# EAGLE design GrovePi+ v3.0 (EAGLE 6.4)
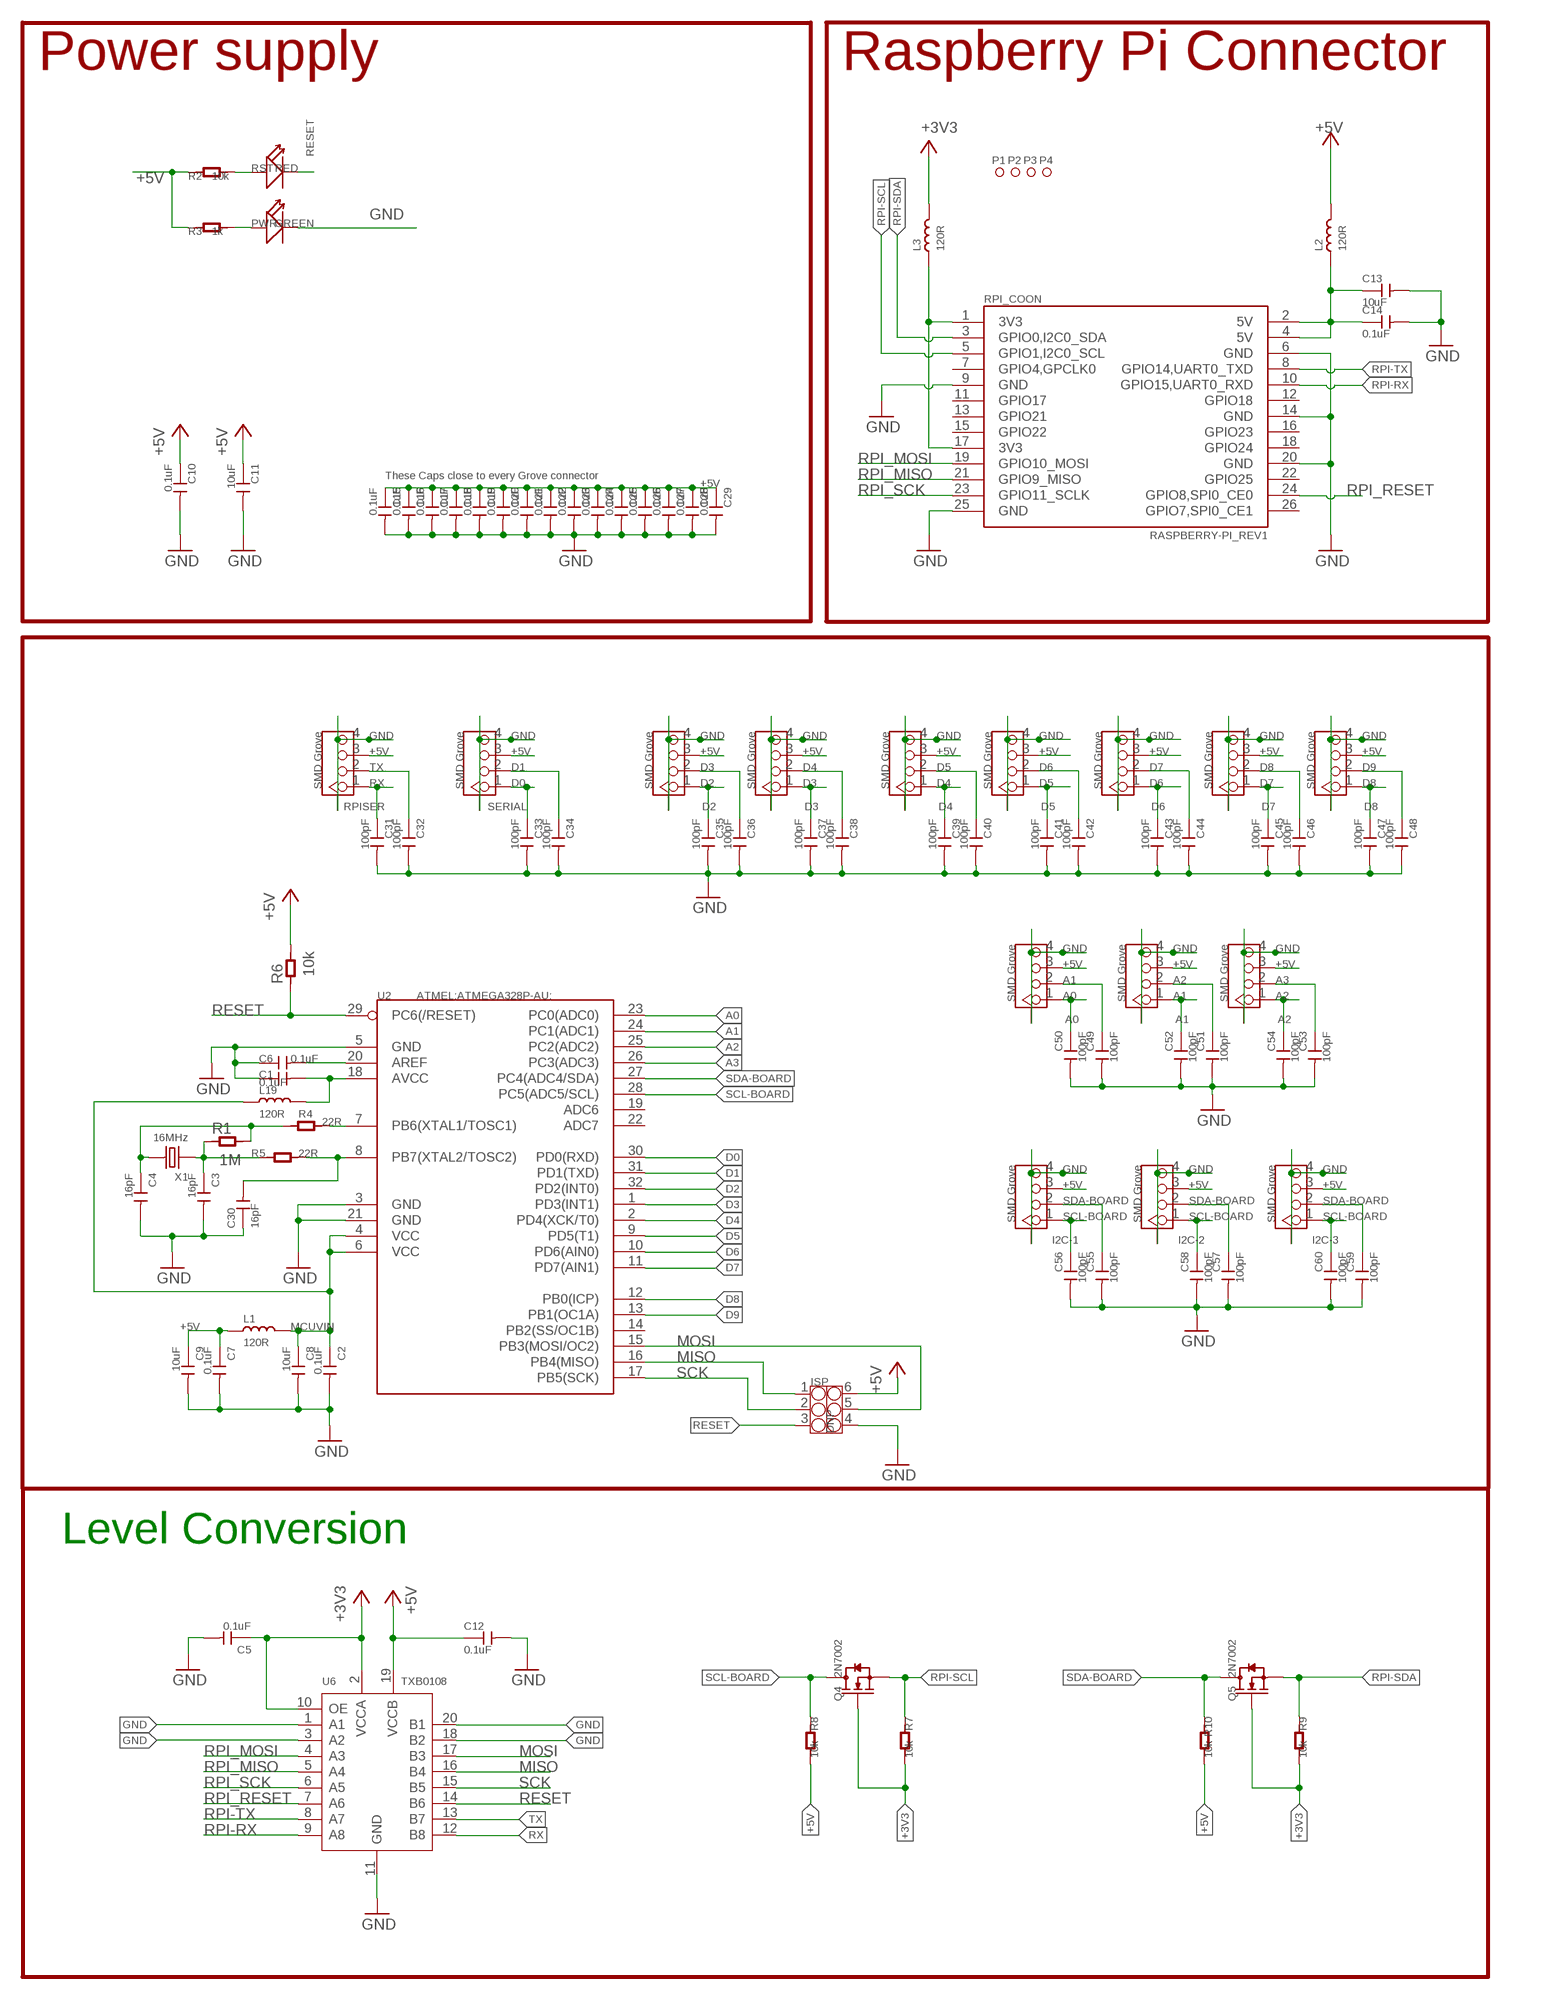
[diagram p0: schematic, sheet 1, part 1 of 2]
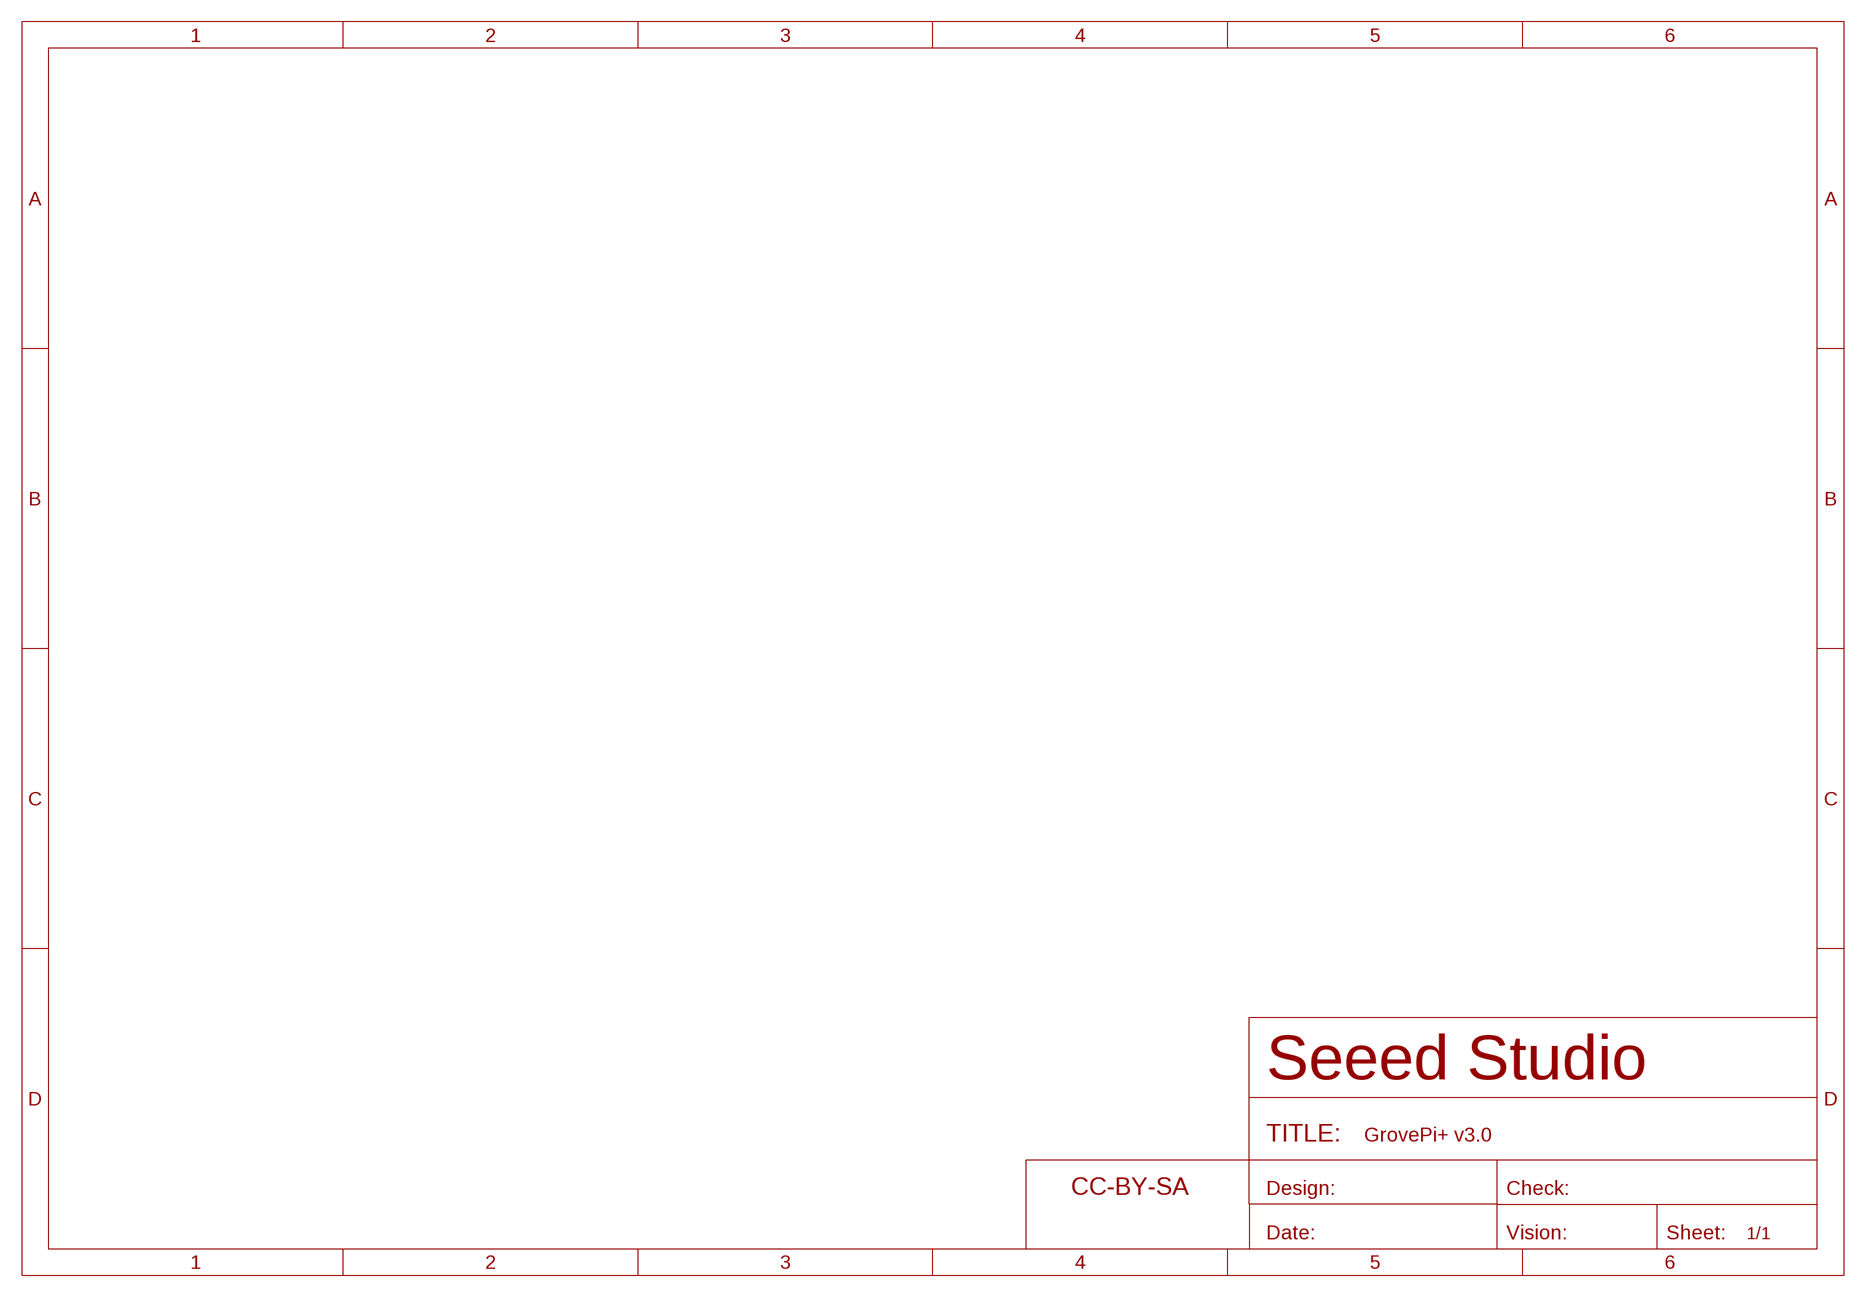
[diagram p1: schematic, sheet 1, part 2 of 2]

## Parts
A0  SMD Grove  GROVE-CONNECTOR-SMD'90D'  [HW4-SMD-2.0-90D]
A1  SMD Grove  GROVE-CONNECTOR-SMD'90D'  [HW4-SMD-2.0-90D]
A2  SMD Grove  GROVE-CONNECTOR-SMD'90D'  [HW4-SMD-2.0-90D]
C1  0.1uF  CAP-0603  [C0603]
C2  0.1uF  CAP-0603  [C0603]
C3  16pF  CAP-0603  [C0603]
C4  16pF  CAP-0603  [C0603]
C5  0.1uF  CAP-0603  [C0603]
C6  0.1uF  CAP-0603  [C0603]
C7  0.1uF  CAP-0603  [C0603]
C8  10uF  CAP-0805  [C0805]
C9  10uF  CAP-0805  [C0805]
C10  0.1uF  CAP-0603  [C0603]
C11  10uF  CAP-0805  [C0805]
C12  0.1uF  CAP-0603  [C0603]
C13  10uF  CAP-0805  [C0805]
C14  0.1uF  CAP-0603  [C0603]
C15  0.1uF  CAP-0603  [C0603]
C16  0.1uF  CAP-0603  [C0603]
C17  0.1uF  CAP-0603  [C0603]
C18  0.1uF  CAP-0603  [C0603]
C19  0.1uF  CAP-0603  [C0603]
C20  0.1uF  CAP-0603  [C0603]
C21  0.1uF  CAP-0603  [C0603]
C22  0.1uF  CAP-0603  [C0603]
C23  0.1uF  CAP-0603  [C0603]
C24  0.1uF  CAP-0603  [C0603]
C25  0.1uF  CAP-0603  [C0603]
C26  0.1uF  CAP-0603  [C0603]
C27  0.1uF  CAP-0603  [C0603]
C28  0.1uF  CAP-0603  [C0603]
C29  0.1uF  CAP-0603  [C0603]
C30  16pF  CAP-0402  [C0402]
C31  100pF  CAP-0603  [C0603]
C32  100pF  CAP-0603  [C0603]
C33  100pF  CAP-0603  [C0603]
C34  100pF  CAP-0603  [C0603]
C35  100pF  CAP-0603  [C0603]
C36  100pF  CAP-0603  [C0603]
C37  100pF  CAP-0603  [C0603]
C38  100pF  CAP-0603  [C0603]
C39  100pF  CAP-0603  [C0603]
C40  100pF  CAP-0603  [C0603]
C41  100pF  CAP-0603  [C0603]
C42  100pF  CAP-0603  [C0603]
C43  100pF  CAP-0603  [C0603]
C44  100pF  CAP-0603  [C0603]
C45  100pF  CAP-0603  [C0603]
C46  100pF  CAP-0603  [C0603]
C47  100pF  CAP-0603  [C0603]
C48  100pF  CAP-0603  [C0603]
C49  100pF  CAP-0603  [C0603]
C50  100pF  CAP-0603  [C0603]
C51  100pF  CAP-0603  [C0603]
C52  100pF  CAP-0603  [C0603]
C53  100pF  CAP-0603  [C0603]
C54  100pF  CAP-0603  [C0603]
C55  100pF  CAP-0603  [C0603]
C56  100pF  CAP-0603  [C0603]
C57  100pF  CAP-0603  [C0603]
C58  100pF  CAP-0603  [C0603]
C59  100pF  CAP-0603  [C0603]
C60  100pF  CAP-0603  [C0603]
D2  SMD Grove  GROVE-CONNECTOR-SMD'90D'  [HW4-SMD-2.0-90D]
D3  SMD Grove  GROVE-CONNECTOR-SMD'90D'  [HW4-SMD-2.0-90D]
D4  SMD Grove  GROVE-CONNECTOR-SMD'90D'  [HW4-SMD-2.0-90D]
D5  SMD Grove  GROVE-CONNECTOR-SMD'DD'  [HW4-SMD-2.0]
D6  SMD Grove  GROVE-CONNECTOR-SMD'DD'  [HW4-SMD-2.0]
D7  SMD Grove  GROVE-CONNECTOR-SMD'90D'  [HW4-SMD-2.0-90D]
D8  SMD Grove  GROVE-CONNECTOR-SMD'90D'  [HW4-SMD-2.0-90D]
I2C-1  SMD Grove  GROVE-CONNECTOR-SMD'90D'  [HW4-SMD-2.0-90D]
I2C-2  SMD Grove  GROVE-CONNECTOR-SMD'90D'  [HW4-SMD-2.0-90D]
I2C-3  SMD Grove  GROVE-CONNECTOR-SMD'90D'  [HW4-SMD-2.0-90D]
ISP  DNP  CONNECTOR-HEADER-2X3P-3460180P1  [2X3P-2.54-2.54-11.6-3.0-BLACK-MALE]
L1  120R  INDUCTOR/FERRITE-BEAD'0603'  [L0603]
L2  120R  INDUCTOR/FERRITE-BEAD'0603'  [L0603]
L3  120R  INDUCTOR/FERRITE-BEAD'0603'  [L0603]
L19  120R  INDUCTOR/FERRITE-BEAD'0603'  [L0603]
P1  PAD-MARK'ANNULAR'  [ROUND-MARK-1.0]
P2  PAD-MARK'ANNULAR'  [ROUND-MARK-1.0]
P3  PAD-MARK'ANNULAR'  [ROUND-MARK-1.0]
P4  PAD-MARK'ANNULAR'  [ROUND-MARK-1.0]
PWR  GREEN  LED  [LED0603]
Q4  2N7002  MOSFET-N-''  [SOT23]
Q5  2N7002  MOSFET-N-''  [SOT23]
R1  1M  R-0402  [R0402]
R2  10k  R-0603  [R0603]
R3  1k  R-0603  [R0603]
R4  22R  R-0402  [R0402]
R5  22R  R-0402  [R0402]
R6  10k  R-0603  [R0603]
R7  10k  R-0603  [R0603]
R8  10k  R-0603  [R0603]
R9  10k  R-0603  [R0603]
R10  10k  R-0603  [R0603]
RPI_COON  RASPBERRY-PI_REV1  [RASPBERRY-PI_REV1]
RPISER  SMD Grove  GROVE-CONNECTOR-SMD'90D'  [HW4-SMD-2.0-90D]
RST  RED  LED  [LED0603]
SERIAL  SMD Grove  GROVE-CONNECTOR-SMD'90D'  [HW4-SMD-2.0-90D]
U2  ATMEL;ATMEGA328P-AU;  ATMEGA328P-AU-1030060P1  [TQFP32]
U6  TXB0108  TXS0108E  [TSSOP20]
U$4  SEEEDSTUDIO-OPEN-SCH-FRAME  [SEEEDSTUDIO-PCB-FRAME]
X1  16MHz  CRYSTAL-2P'5032'  [X2-SMD-5.0X3.2X1.3MM]

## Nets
+3V3: C5.1 L3.2 Q4.1(G) Q5.1(G) R7.2 R9.2 U6.2(VCCA) U6.10(OE)
+5V: A0.3 A1.3 A2.3 C7.1 C9.1 C10.1 C11.1 C12.1 C15.1 C16.1 C17.1 C18.1 C19.1 C20.1 C21.1 C22.1 C23.1 C24.1 C25.1 C26.1 C27.1 C28.1 C29.1 D2.3 D3.3 D4.3 D5.3 D6.3 D7.3 D8.3 I2C-1.3 I2C-2.3 I2C-3.3 ISP.6 L1.1 L2.2 R2.1 R3.1 R6.2 R8.2 R10.2 RPISER.3 SERIAL.3 U6.19(VCCB)
A0: A0.1 C50.1 U2.23(PC0(ADC0))
A1: A0.2 A1.1 C49.1 C52.1 U2.24(PC1(ADC1))
A2: A1.2 A2.1 C51.1 C54.1 U2.25(PC2(ADC2))
A3: A2.2 C53.1 U2.26(PC3(ADC3))
D0: C33.1 SERIAL.1 U2.30(PD0(RXD))
D1: C34.1 SERIAL.2 U2.31(PD1(TXD))
D2: C35.1 D2.1 U2.32(PD2(INT0))
D3: C36.1 C37.1 D2.2 D3.1 U2.1(PD3(INT1))
D4: C38.1 C39.1 D3.2 D4.1 U2.2(PD4(XCK/T0))
D5: C40.1 C41.1 D4.2 D5.1 U2.9(PD5(T1))
D6: C42.1 C43.1 D5.2 D6.1 U2.10(PD6(AIN0))
D7: C44.1 C45.1 D6.2 D7.1 U2.11(PD7(AIN1))
D8: C46.1 C47.1 D7.2 D8.1 U2.12(PB0(ICP))
D9: C48.1 D8.2 U2.13(PB1(OC1A))
GND: A0.4 A0.SS1 A0.SS2 A1.4 A1.SS1 A1.SS2 A2.4 A2.SS1 A2.SS2 C1.1 C2.2 C3.2 C4.2 C5.2 C6.1 C7.2 C8.2 C9.2 C10.2 C11.2 C12.2 C13.2 C14.2 C15.2 C16.2 C17.2 C18.2 C19.2 C20.2 C21.2 C22.2 C23.2 C24.2 C25.2 C26.2 C27.2 C28.2 C29.2 C30.1 C31.2 C32.2 C33.2 C34.2 C35.2 C36.2 C37.2 C38.2 C39.2 C40.2 C41.2 C42.2 C43.2 C44.2 C45.2 C46.2 C47.2 C48.2 C49.2 C50.2 C51.2 C52.2 C53.2 C54.2 C55.2 C56.2 C57.2 C58.2 C59.2 C60.2 D2.4 D2.SS1 D2.SS2 D3.4 D3.SS1 D3.SS2 D4.4 D4.SS1 D4.SS2 D5.4 D5.SS1 D5.SS2 D6.4 D6.SS1 D6.SS2 D7.4 D7.SS1 D7.SS2 D8.4 D8.SS1 D8.SS2 I2C-1.4 I2C-1.SS1 I2C-1.SS2 I2C-2.4 I2C-2.SS1 I2C-2.SS2 I2C-3.4 I2C-3.SS1 I2C-3.SS2 ISP.4 PWR.- RPI_COON.6(GND) RPI_COON.9(GND) RPI_COON.14(GND) RPI_COON.20(GND) RPI_COON.25(GND) RPISER.4 RPISER.SS1 RPISER.SS2 SERIAL.4 SERIAL.SS1 SERIAL.SS2 U2.3(GND) U2.5(GND) U2.21(GND) U6.1(A1) U6.3(A2) U6.11(GND) U6.18(B2) U6.20(B1)
MCUVIN: C2.1 C8.1 L1.2 L19.1 U2.4(VCC) U2.6(VCC)
MISO: ISP.1 U2.16(PB4(MISO)) U6.16(B4)
MOSI: ISP.5 U2.15(PB3(MOSI/OC2)) U6.17(B3)
N$1: C3.1 R1.1 R5.1 X1.1
N$2: PWR.+ R3.2
N$3: C4.1 R1.2 R4.1 X1.2
N$4: C1.2 L19.2 U2.18(AVCC)
N$17: R2.2 RST.+
N$19: L3.1 RPI_COON.1(3V3) RPI_COON.17(3V3)
N$20: C6.2 U2.20(AREF)
N$21: C13.1 C14.1 L2.1 RPI_COON.2(5V) RPI_COON.4(5V)
N$22: C30.2 R5.2 U2.8(PB7(XTAL2/TOSC2))
N$23: R4.2 U2.7(PB6(XTAL1/TOSC1))
RESET: ISP.3 R6.1 RST.- U2.29(PC6(/RESET)) U6.14(B6)
RPI-RX: RPI_COON.10(GPIO15,UART0_RXD) U6.9(A8)
RPI-SCL: Q4.2(S) R7.1 RPI_COON.5(GPIO1,I2C0_SCL)
RPI-SDA: Q5.2(S) R9.1 RPI_COON.3(GPIO0,I2C0_SDA)
RPI-TX: RPI_COON.8(GPIO14,UART0_TXD) U6.8(A7)
RPI_MISO: RPI_COON.21(GPIO9_MISO) U6.5(A4)
RPI_MOSI: RPI_COON.19(GPIO10_MOSI) U6.4(A3)
RPI_RESET: RPI_COON.24(GPIO8,SPI0_CE0) U6.7(A6)
RPI_SCK: RPI_COON.23(GPIO11_SCLK) U6.6(A5)
RX: C31.1 RPISER.1 U6.12(B8)
SCK: ISP.2 U2.17(PB5(SCK)) U6.15(B5)
SCL-BOARD: C56.1 C58.1 C60.1 I2C-1.1 I2C-2.1 I2C-3.1 Q4.3(D) R8.1 U2.28(PC5(ADC5/SCL))
SDA-BOARD: C55.1 C57.1 C59.1 I2C-1.2 I2C-2.2 I2C-3.2 Q5.3(D) R10.1 U2.27(PC4(ADC4/SDA))
TX: C32.1 RPISER.2 U6.13(B7)
Unconnected: RPI_COON.7(GPIO4,GPCLK0) RPI_COON.11(GPIO17) RPI_COON.12(GPIO18) RPI_COON.13(GPIO21) RPI_COON.15(GPIO22) RPI_COON.16(GPIO23) RPI_COON.18(GPIO24) RPI_COON.22(GPIO25) RPI_COON.26(GPIO7,SPI0_CE1) U2.14(PB2(SS/OC1B)) U2.19(ADC6) U2.22(ADC7)

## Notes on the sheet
- Power supply | Raspberry Pi Connector
- These Caps close to every Grove connector
- Level Conversion

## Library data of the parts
A0 A1 A2 D2-D8 I2C-1-I2C-3 RPISER SERIAL = Connector-new:GROVE-CONNECTOR-SMD: 4P-SMD-2.0:320110030;4P-SMD-2.0-90D:320110032
C1-C60 = OPL:CAP: Ceramic Capacitors
ISP = OPL:CONNECTOR-HEADER-2X3P
L1-L3 L19 = Discrete-new:INDUCTOR/FERRITE-BEAD
P1-P4 = Discrete-new:PAD-MARK; PARTNO: DNP
PWR RST = OPL:LED*: LED
Q4 Q5 = OPL:MOSFET-N: CJ2302：SMD MOSFET N-CH 20V-2.1A
R1-R10 = OPL:R*
RPI_COON = RaspberryPi:RASPBERRY-PI_REV1: Raspberry Pi Board Jacques Lagnel V1.0 (beta) 2012 Mateusz Bawaj V1.1 (beta) 2012 Board dimension: Forum 3D model The GPIO Connector (P1): http://elinux.org/RPi_Low-level_peripherals
U2 = OPL:ATMEGA328P-AU: 8-bit AVR Microcontroller with 32K Bytes In-System Programmable Flash
U6 = template:TXS0108E: 8-BIT BIDIRECTIONAL VOLTAGE-LEVEL TRANSLATOR FOR OPEN-DRAIN AND PUSH-PULL APPLICATIONS
U$4 = moudle-new:SEEEDSTUDIO-OPEN-SCH-FRAME
X1 = Discrete-new:CRYSTAL-2P

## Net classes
0 default: width 0.203 mm
2 POWER: width 0.152 mm, drill 0.356 mm, clearance 0.051 mm

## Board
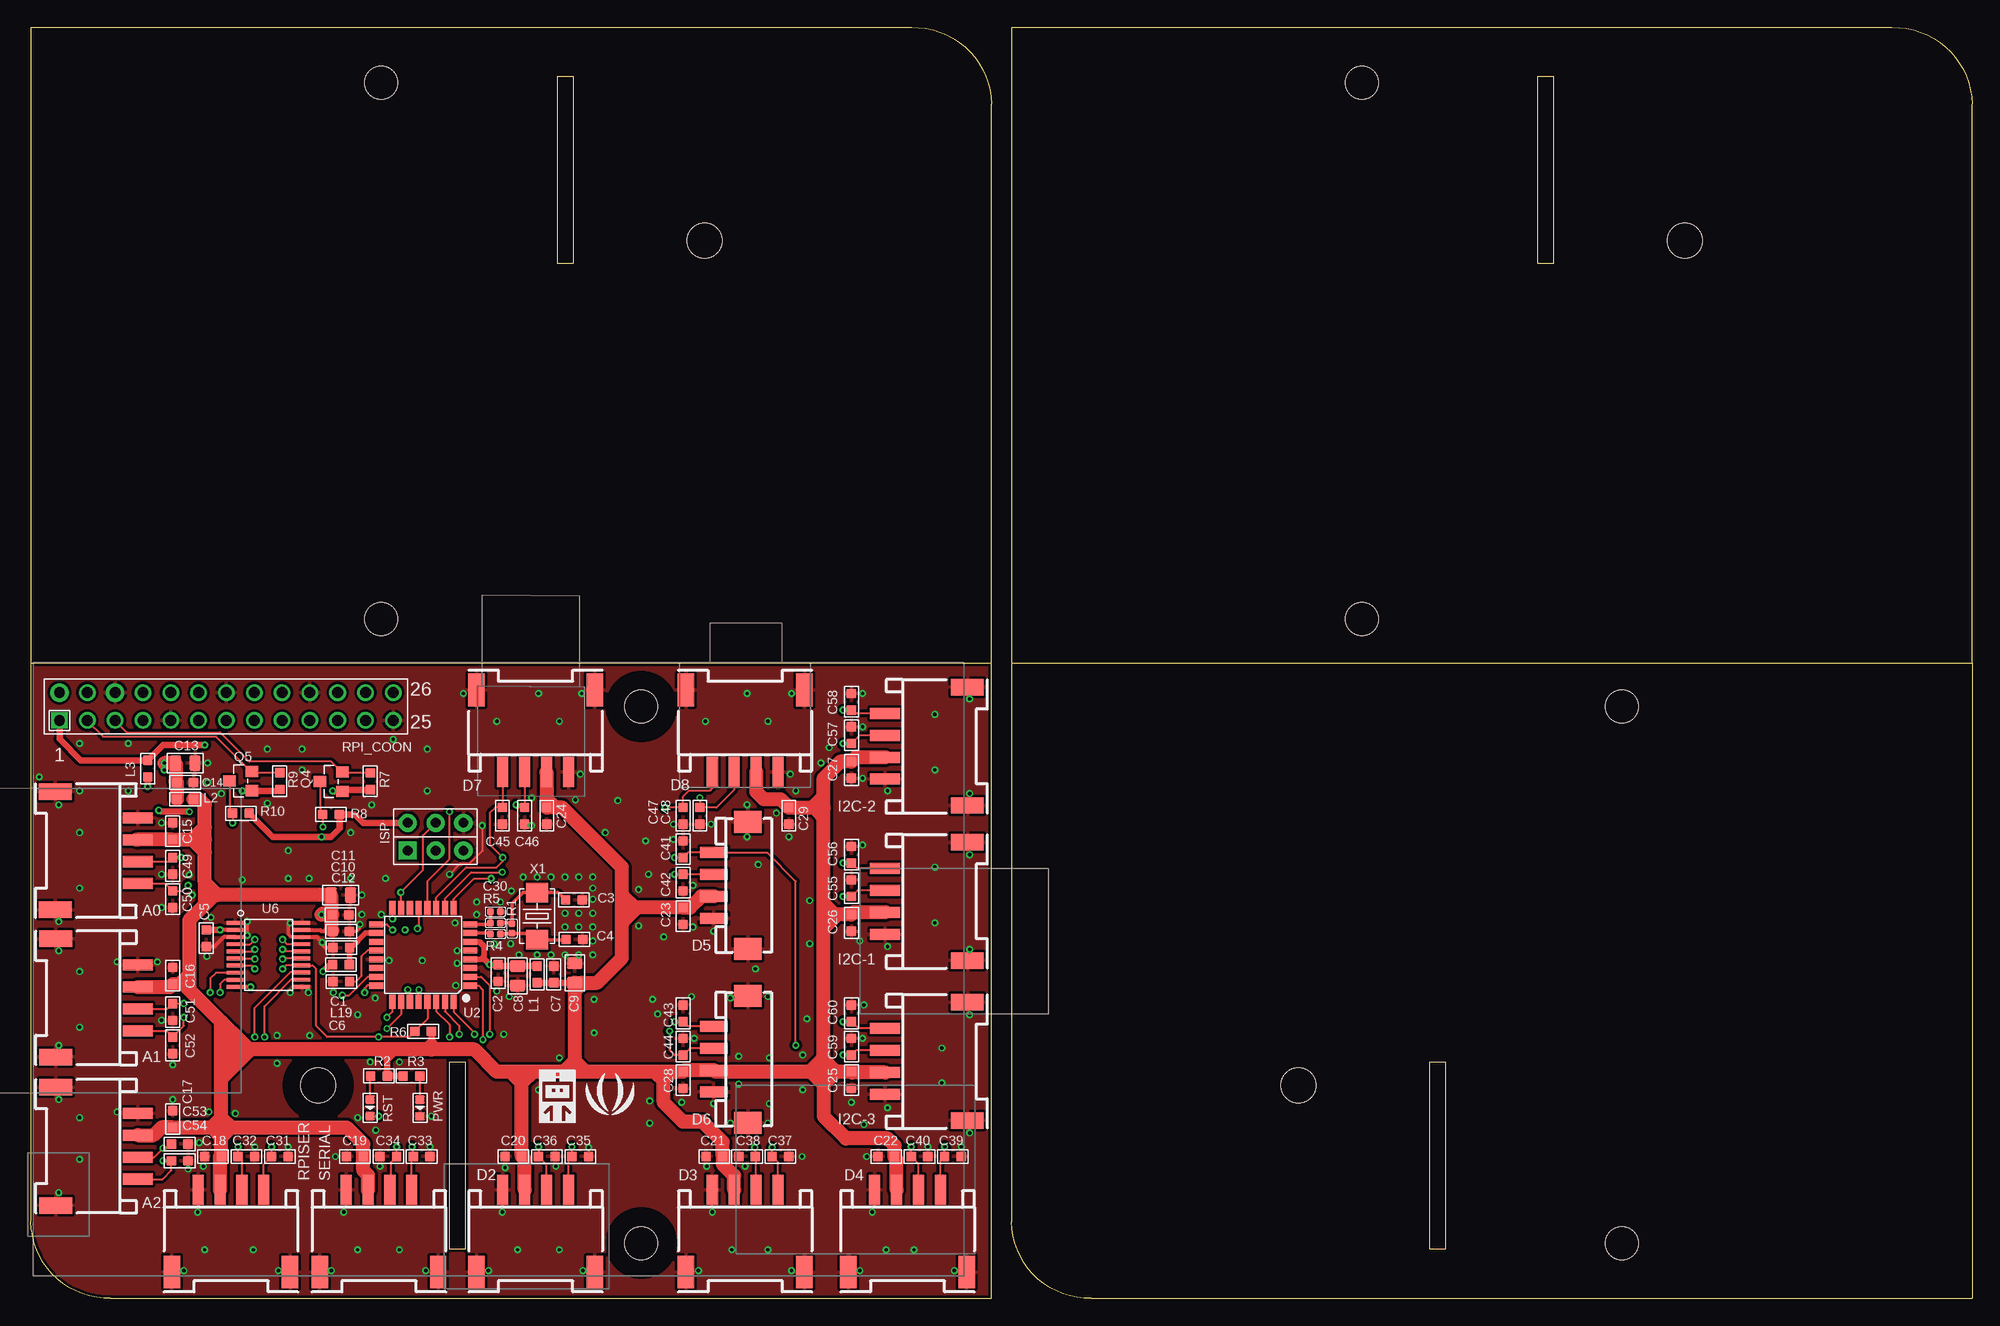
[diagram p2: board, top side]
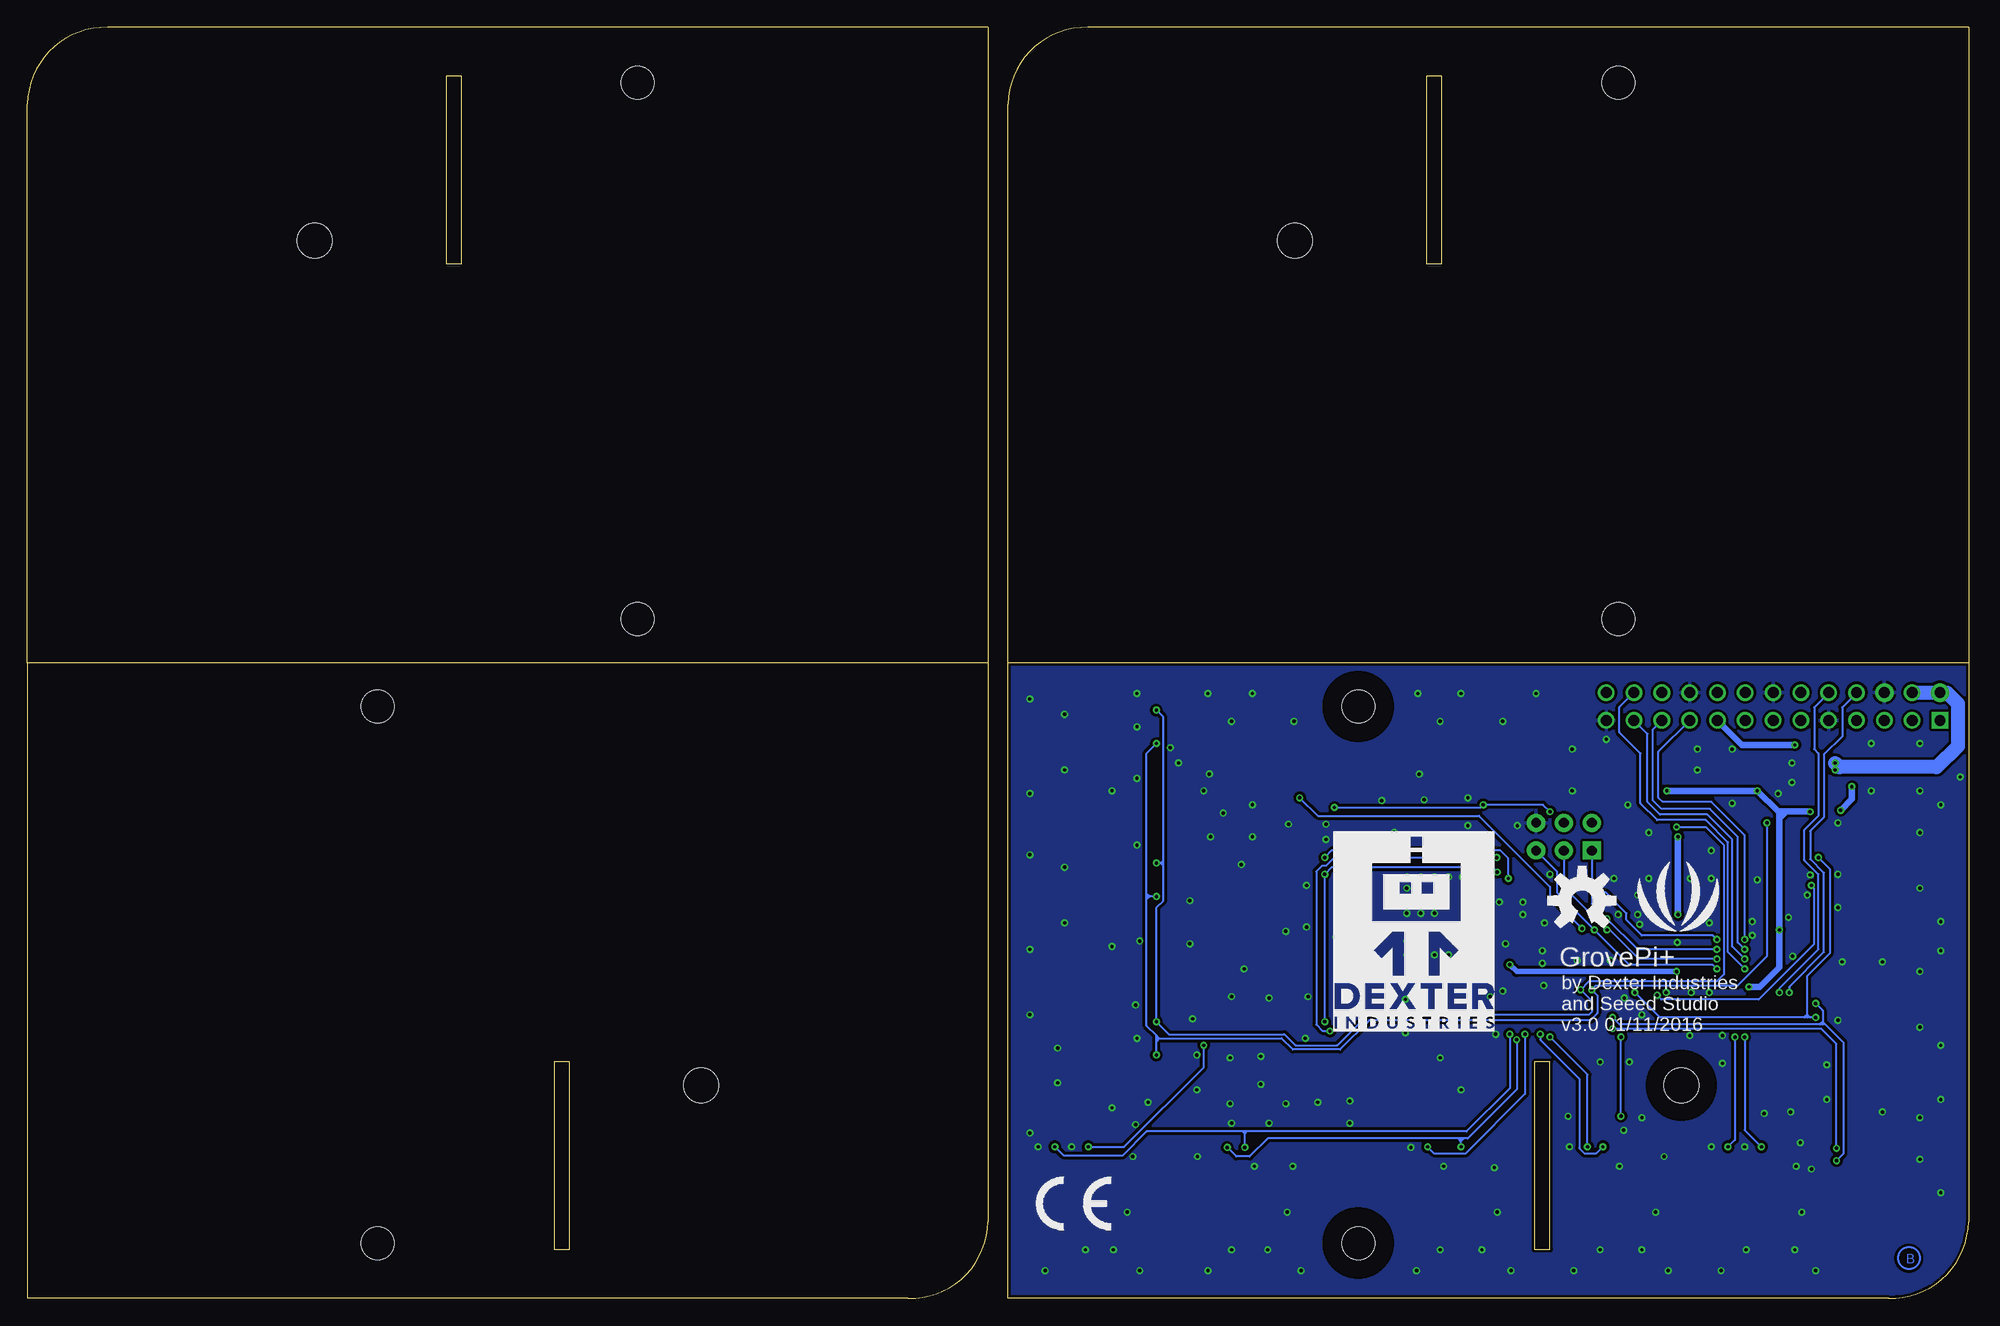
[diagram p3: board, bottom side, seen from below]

Size 177.27 x 116.08 mm. Coordinates in mm from the lower left corner, seen from the top.
Outline: 87.73,58.04 87.73,0 7.32,0 arc-90 0,7.01 0,58.04
Outline: 89.53,58.04 177.27,58.04
Outline: 177.27,58.04 177.27,109.07 arc90 169.95,116.08 89.53,116.08 89.53,58.04
Outline: 0,58.04 0,116.08 80.42,116.08 arc-90 87.73,109.07 87.73,58.04
Outline: 0,58.04 87.73,58.04
Outline: 89.53,58.04 89.53,7.01 arc90 96.85,0 177.27,0 177.27,58.04
Outline: 38.23,21.59 39.65,21.59 39.65,4.47 38.23,4.47 38.23,21.59
Outline: 139.04,94.49 137.62,94.49 137.62,111.61 139.04,111.61 139.04,94.49
Outline: 49.51,94.49 48.08,94.49 48.08,111.61 49.51,111.61 49.51,94.49
Outline: 127.76,21.59 129.18,21.59 129.18,4.47 127.76,4.47 127.76,21.59
Copper layers (1*16): Top 0.035mm / dielectric 1.5mm / Bottom 0.035mm
Design rules "SeeedStudio_2layer_DRU_no_angle_20140221 *": minimum track width 6mil, minimum drill 12mil, track to track 6mil, track to pad 6mil, pad to pad 6mil, via to via 6mil, smd to smd 0mil, copper to edge 10mil, drill to drill 10mil, minimum pad ring 10mil, minimum via ring 6mil, stop-mask expansion 2mil, vias tented up to drill 25mil, thermal gap 10mil
Holes 3.2 mm at 26.23,19.46 151.04,96.62 61.51,96.62 115.76,19.46
Holes 3 mm at 55.73,54.05 55.73,5.05 121.53,62.03 121.53,111.03 32,62.03 32,111.03 145.27,54.05 145.27,5.05
Holes 2.03 mm at 2.54,-4.45 2.54,120.65 174.62,120.65 174.65,-4.45
tRestrict: area 23.2,16.5 to 29.2,22.5; area 52.7,2 to 58.7,8; area 52.7,51.1 to 58.7,57.1
bRestrict: area 52.7,2 to 58.7,8; area 23.2,16.5 to 29.2,22.5; area 52.7,51.1 to 58.7,57.1

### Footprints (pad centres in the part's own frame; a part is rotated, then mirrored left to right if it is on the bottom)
HW4-SMD-2.0-90D = smd 1.01 x 2.74: 1 -3,-0.1; 2 -1,-0.1; 3 1,-0.1; 4 3,-0.1 | smd 1.5 x 3: SS1 -5.4,7.4; SS2 5.4,7.4
C0603 = smd 0.889 x 0.889: 1 -0.762,0; 2 0.762,0
C0805 = smd 1.016 x 1.397: 1 -0.889,0; 2 0.889,0
C0402 = smd 0.635 x 0.635: 1 -0.445,0; 2 0.445,0
HW4-SMD-2.0 = smd 1 x 2.5: 1 -3,0; 2 -1,0; 3 1,0; 4 3,0 | smd 2 x 2.5: SS1 -5.8,3.123; SS2 5.8,3.123
2X3P-2.54-2.54-11.6-3.0-BLACK-MALE = drill 0.889 pad 1.651 square: 1 -1.27,2.54 | drill 0.889 pad 1.651: 2 -1.27,0; 3 -1.27,-2.54; 4 1.27,-2.54; 5 1.27,0; 6 1.27,2.54
L0603 = smd 0.889 x 0.889: 1 -0.762,0; 2 0.762,0
ROUND-MARK-1.0 = smd 1.016 x 1.016: P$1 0,0
LED0603 = smd 0.762 x 0.889: + -0.762,0; - 0.762,0
SOT23 = smd 1.016 x 1.143: 1 -0.889,-1.016; 2 0.889,-1.016; 3 0,1.016
R0402 = smd 0.635 x 0.635: 1 -0.445,0; 2 0.445,0
R0603 = smd 0.889 x 0.889: 1 -0.762,0; 2 0.762,0
RASPBERRY-PI_REV1 = drill 1 square: 1 -41.91,21.59 | drill 1 pad 1.676: 2 -41.91,24.13; 6 -36.83,24.13 | drill 1: 3 -39.37,21.59; 4 -39.37,24.13; 5 -36.83,21.59; 7 -34.29,21.59; 8 -34.29,24.13; 9 -31.75,21.59; 10 -31.75,24.13; 11 -29.21,21.59; 12 -29.21,24.13; 13 -26.67,21.59; 14 -26.67,24.13; 15 -24.13,21.59; 16 -24.13,24.13; 17 -21.59,21.59; 18 -21.59,24.13; 19 -19.05,21.59; 20 -19.05,24.13; 21 -16.51,21.59; 22 -16.51,24.13; 23 -13.97,21.59; 24 -13.97,24.13; 25 -11.43,21.59; 26 -11.43,24.13
TQFP32 = smd 1.27 x 0.559: 1 -4.293,2.8; 2 -4.293,2; 3 -4.293,1.2; 4 -4.293,0.4; 5 -4.293,-0.4; 6 -4.293,-1.2; 7 -4.293,-2; 8 -4.293,-2.8; 17 4.293,-2.8; 18 4.293,-2; 19 4.293,-1.2; 20 4.293,-0.4; 21 4.293,0.4; 22 4.293,1.2; 23 4.293,2; 24 4.293,2.8 | smd 0.559 x 1.27: 9 -2.8,-4.293; 10 -2,-4.293; 11 -1.2,-4.293; 12 -0.4,-4.293; 13 0.4,-4.293; 14 1.2,-4.293; 15 2,-4.293; 16 2.8,-4.293; 25 2.8,4.293; 26 2,4.293; 27 1.2,4.293; 28 0.4,4.293; 29 -0.4,4.293; 30 -1.2,4.293; 31 -2,4.293; 32 -2.8,4.293
TSSOP20 = smd 0.35 x 1.5: 1 -2.925,-3.065; 2 -2.275,-3.065; 3 -1.625,-3.065; 4 -0.975,-3.065; 5 -0.325,-3.065; 6 0.325,-3.065; 7 0.975,-3.065; 8 1.625,-3.065; 9 2.275,-3.065; 10 2.925,-3.065; 11 2.91,3.065; 12 2.26,3.065; 13 1.61,3.065; 14 0.96,3.065; 15 0.325,3.065; 16 -0.325,3.065; 17 -0.975,3.065; 18 -1.625,3.065; 19 -2.275,3.065; 20 -2.925,3.065
X2-SMD-5.0X3.2X1.3MM = smd 1.778 x 2.032: 1 -2.159,0; 2 2.159,0

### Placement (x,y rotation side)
A0  9.64,40.88 90 top
A1  9.67,27.44 90 top
A2  9.66,13.9 90 top
C1  28.35,32.03 0 top
C2  42.67,29.72 270 top
C3  49.59,36.39 0 top
C4  49.63,32.79 0 top
C5  16.03,32.89 270 top
C6  28.35,28.93 0 top
C7  47.75,29.59 90 top
C8  44.45,29.46 270 top
C9  49.66,29.72 90 top
C10  28.29,35.03 0 top
C11  28.3,36.83 0 top
C12  28.33,33.52 0 top
C13  14.1,48.9 0 top
C14  14.1,47.12 0 top
C15  12.95,42.67 90 top
C16  12.95,29.46 90 top
C17  12.95,16.38 90 top
C18  16.64,12.95 180 top
C19  29.59,12.95 180 top
C20  44.07,12.95 180 top
C21  62.42,12.95 180 top
C22  78.11,12.95 180 top
C23  59.56,34.92 270 top
C24  47.12,44.07 270 top
C25  74.93,19.94 270 top
C26  74.93,34.29 270 top
C27  74.93,48.26 270 top
C28  59.56,19.94 270 top
C29  69.22,44.07 270 top
C30  42.42,35.31 180 top
C31  22.73,12.95 0 top
C32  19.68,12.95 0 top
C33  35.69,12.95 0 top
C34  32.64,12.95 180 top
C35  50.16,12.95 0 top
C36  47.12,12.95 0 top
C37  68.45,12.95 0 top
C38  65.41,12.95 180 top
C39  84.2,12.95 0 top
C40  81.15,12.95 0 top
C41  59.56,41.02 90 top
C42  59.56,37.97 270 top
C43  59.56,26.04 90 top
C44  59.56,22.99 90 top
C45  43.05,44.07 270 top
C46  45.09,44.07 270 top
C47  59.56,44.07 270 top
C48  61.09,44.07 270 top
C49  12.95,39.5 270 top
C50  12.95,36.45 270 top
C51  12.95,26.16 270 top
C52  12.95,23.11 270 top
C53  13.59,14.1 0 top
C54  13.59,12.57 0 top
C55  74.93,37.47 90 top
C56  74.93,40.51 90 top
C57  74.93,51.44 90 top
C58  74.93,54.48 90 top
C59  74.93,22.99 90 top
C60  74.93,26.04 90 top
D2  46.09,9.8 180 top
D3  65.23,9.8 180 top
D4  80.05,9.8 180 top
D5  62.36,37.72 270 top
D6  62.36,21.84 270 top
D7  46.09,48.18 0 top
D8  65.23,48.18 0 top
I2C-1  78.11,36.26 270 top
I2C-2  78.11,50.42 270 top
I2C-3  78.11,21.64 270 top
ISP  36.96,42.16 90 top
L1  46.23,29.59 90 top
L2  14.1,45.59 0 top
L3  10.67,48.39 270 top
L19  28.32,30.48 0 top
P1  not placed on the board
P2  not placed on the board
P3  not placed on the board
P4  not placed on the board
PWR  35.53,17.4 270 top
Q4  27.42,47.2 90 top
Q5  19.17,47.25 90 top
R1  43.94,33.78 270 top
R2  31.8,20.31 180 top
R3  34.76,20.31 0 top
R4  42.42,33.27 180 top
R5  42.42,34.29 180 top
R6  35.82,24.39 0 top
R7  31,47.22 270 top
R8  27.42,44.2 0 top
R9  22.73,47.24 270 top
R10  19.17,44.3 0 top
RPI_COON  44.53,31.19 0 top
RPISER  18.28,9.8 180 top
RST  30.97,17.41 270 top
SERIAL  31.79,9.8 180 top
U2  35.81,31.37 180 top
U6  21.7,31.37 270 top
U$1  [OSHW_FILLX250_NOTEXT]  35.31,36.32 0 bottom
U$2  [SEEED_LOGO250]  30.23,33.53 0 bottom
U$3  [SEEED-LOGO-150]  50.67,16.76 0 top
U$4  not placed on the board
X1  46.23,34.91 270 top

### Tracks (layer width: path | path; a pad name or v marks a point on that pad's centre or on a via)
+3V3  (via drill 0.3 pad 0.64)
  Top 0.356: C5.1 | U6.2 17.28,33.65 v17.27,33.66
  Top 0.406: U6.10 v20.07,28.45 | v20.07,28.45
  Top 0.61: R9.2 22.62,46.36 Q5.1 19.31,46.36 v19.3,46.35 | R7.2 28.58,46.46 Q4.1 27.61,46.31 v27.56,46.35 | C5.1 v17.27,33.65 v17.27,33.66 | v11.68,44.58 11.81,44.45 v14.48,44.45 | L3.2 v10.67,46.74
  Bottom 0.61: v27.56,46.35 v19.3,46.35 17.4,44.45 | 17.4,44.45 17.27,44.32 17.27,43.81 | 17.27,43.81 v17.27,33.66 17.27,30.23 19.05,28.45 v20.07,28.45 | v20.07,28.45 | v11.68,44.58 10.67,45.59 v10.67,46.74 | v14.48,44.45 16.64,44.45 | 16.64,44.45 17.4,44.45 | 16.64,44.45 17.27,43.81
+5V  (via drill 0.3 pad 0.64)
  Top 0.356: U6.19 26.42,33.65 26.55,33.52 C12.1
  Top 0.61: 27.52,33.57 C12.1 | ISP.6 30.35,43.43 29.59,44.2 R8.2 28.18,42.91 27.43,42.16 v26.54,42.16 22.07,42.16 R10.2 | R2.1 R3.1 | 32.64,20.23 R2.1 | 62.56,20.64 D6.3 | R2.1 32.56,21.76 | 32.56,21.8 32.56,22.65 32.64,22.73 | 35.05,22.74 35.05,22.73 | 32.56,21.8 32,22.35 | 32.56,21.76 33.15,22.35 | 32.56,21.76 32.56,21.8 | C9.1 C7.1 L1.1 46.1,28.83 | R6.2 36.58,23.63 | 36.58,23.62 36.58,22.74 36.58,22.73 | 36.58,23.63 35.94,22.99 | 36.58,23.63 36.58,23.62 | 36.58,23.62 37.21,22.99
  Top 1.27: 27.41,35.14 C11.1 17.02,36.83 | 27.41,35.14 C10.1 | 27.41,35.14 27.41,33.68 27.52,33.57 | 27.41,35.14 26.63,35.14 v26.54,35.05 | 16.77,36.83 16,36.83 15.88,36.96 | 15.88,37.97 15.88,36.96 | 15.88,36.96 15.88,35.94 14.48,34.54 14.48,28.7 | 17.02,36.83 16.77,36.83 | 16.77,36.83 16,36.07 | 17.02,36.83 15.88,37.97 | A1.3 12.69,28.44 C16.1 13.59,28.7 | 20.07,22.73 32.64,22.73 35.05,22.73 36.58,22.73 40.51,22.73 42.55,20.7 44.83,20.7 | 20.07,22.73 19.94,22.73 | D2.3 45.09,12.7 C20.1 44.83,19.68 | I2C-2.3 75.33,49.42 C27.1 73.91,49.02 72.39,47.5 72.39,44.83 | D8.3 66.23,46.3 66.93,45.59 68.45,45.59 C29.1 71.37,44.83 | I2C-1.3 75.14,35.26 C26.1 73.66,35.05 | D4.3 79.05,12.64 78.87,12.83 C22.1 78.87,13.97 78.23,14.61 74.42,14.61 72.39,16.64 72.39,19.56 | 15.88,37.97 15.88,40.77 | 15.88,40.77 15.88,41.91 | 15.88,41.91 15.88,43.05 | 15.88,43.05 15.88,45.09 15.37,45.59 L2.2 | 14.73,41.91 C15.1 9.71,41.91 | 14.73,41.91 15.88,41.91 | 9.65,41.91 9.71,41.91 | 9.71,41.91 A0.3 | 14.73,41.91 15.88,43.05 | 14.73,41.91 15.88,40.77 | 14.48,28.7 14.48,28.19 | 14.48,28.19 17.4,25.27 | 17.4,25.27 19.05,23.62 | 19.05,23.62 19.94,22.73 | 13.59,28.7 13.97,28.7 | 13.97,28.7 14.48,28.7 | 14.48,28.19 13.97,28.7 | 13.59,28.7 14.35,29.46 | A2.3 11.21,14.9 11.94,15.62 C17.1 16.51,15.62 | C18.1 17.4,13.08 | 17.4,13.08 17.4,14.73 | 17.4,14.73 17.4,15.62 | 17.4,15.62 17.4,16.51 | 17.4,16.51 17.4,20.07 | 17.4,20.07 17.4,22.73 | 17.4,22.73 17.4,25.27 | 19.94,22.73 17.4,22.73 | 19.05,23.62 18.29,23.62 18.03,23.37 18.03,21.72 18.16,21.59 | 20.07,22.73 17.4,20.07 | 16.51,15.62 17.4,15.62 | 16.51,15.62 17.27,16.38 | 16.51,15.62 17.4,14.73 | RPISER.3 17.27,12.96 17.4,13.08
  Top 1.27: 17.4,15.62 18.29,15.62 | 18.29,15.62 28.83,15.62 30.35,14.1 C19.1 30.35,11.68 30.79,11.25 SERIAL.3 | 58.55,20.7 C28.1 59.71,20.84 D6.3 62.5,20.7 72.39,20.7 | 58.55,20.7 57.78,20.7 | 57.78,20.7 50.67,20.7 | 50.67,20.7 49.66,20.7 | 49.66,20.7 45.85,20.7 | 45.85,20.7 44.83,20.7 | 49.66,28.07 C9.1 50.42,28.83 | 49.66,28.07 49.66,21.72 | 49.66,21.72 49.66,20.7 | 44.83,19.68 44.83,20.7 | 44.83,19.68 43.94,20.57 | 44.83,19.68 45.85,20.7 | 49.66,21.72 48.77,20.83 | 49.66,21.72 50.67,20.7 | D3.3 64.23,11.21 63.18,12.26 C21.1 63.18,14.28 61.34,16.13 59.55,16.13 57.78,17.89 57.78,19.94 | 57.78,19.94 57.78,20.7 | 57.78,19.94 57.15,20.57 | 57.78,19.94 58.55,20.7 | D5.3 61.23,36.72 60.2,35.69 C23.1 55.37,35.69 | 50.42,28.83 51.69,28.83 53.98,31.11 53.98,35.69 | I2C-3.3 74.99,20.64 C25.1 72.39,20.7 | 72.39,21.84 72.39,20.7 | 72.39,21.97 71.25,20.83 | 72.39,21.97 72.39,21.84 | 72.39,21.84 73.41,20.83 | 72.39,21.97 72.39,35.05 | 72.39,35.05 72.39,36.07 | 72.39,36.07 72.39,44.83 | 73.66,35.05 73.41,35.05 | 73.41,35.05 72.39,35.05 | 73.41,35.05 72.39,36.07 | 73.66,35.05 72.52,33.91 | 71.5,44.83 72.39,44.83 | 71.37,44.83 72.14,45.59 | 71.37,44.83 71.5,44.83 | 71.5,44.83 72.14,44.2 | D7.3 47.09,45.62 | 47.09,45.62 47.09,44.86 C24.1 47.88,44.83 | 72.39,20.7 72.39,19.56 | 72.39,19.56 71.37,20.57 | 72.39,19.56 73.28,20.45 | 47.88,44.83 48.51,44.83 53.98,39.37 53.98,35.69 | 47.09,45.62 47.88,44.83 | 50.42,28.83 49.66,28.07 | 17.4,16.51 18.16,15.75 | 18.29,15.62 17.4,14.73 | 55.12,35.69 53.98,35.69 | 55.37,35.69 55.12,35.69 | 55.12,35.69 54.1,36.7 | 55.37,35.69 54.1,34.42
  Bottom 0.61: v26.54,35.05 v26.54,42.16
A0  (via drill 0.3 pad 0.64)
  Top 0.203: U2.23 30.77,29.37 29.08,27.69 v28.45,27.69 | A0.1 12.28,37.88 C50.1 13.84,37.21 v14.35,37.72
  Bottom 0.203: v28.45,27.69 28.07,27.3 19.18,27.3 14.1,32.38 14.1,37.47 v14.35,37.72
A1  (via drill 0.3 pad 0.64)
  Top 0.203: U2.24 30.73,28.57 30.48,28.32 v30.48,27.94 | C49.1 13.08,40.26 | 13.08,40.26 v13.72,40.26 | v13.97,25.65 13.97,24.89 C52.1 12.39,24.44 A1.1 | A0.2 12.71,39.88 13.08,40.26
  Bottom 0.203: v13.97,25.65 14.48,25.65 | 14.48,25.65 14.73,25.65 | 14.73,25.65 14.99,25.65 | 14.99,25.65 28.19,25.65 v30.48,27.94 | v13.72,40.26 12.7,39.24 12.7,31.5 14.73,29.46 14.73,25.91 | 14.73,25.91 14.73,25.65 | 14.73,25.91 14.48,25.65 | 14.73,25.91 14.99,25.65
A2  (via drill 0.3 pad 0.64)
  Top 0.203: U2.25 33.01,26.16 v32.51,25.65 | v13.97,26.92 C51.1 12.47,26.44 A1.2 | v12.06,12.57 C54.1 12.83,11.68 12.04,10.9 A2.1
  Bottom 0.203: 13.08,25.02 11.43,23.37 11.43,13.21 v12.06,12.57 | 13.08,25.02 13.34,25.02 | 13.34,25.02 13.59,25.02 | 13.59,25.02 31.88,25.02 v32.51,25.65 | v13.97,26.92 13.34,26.29 13.34,25.27 | 13.34,25.27 13.34,25.02 | 13.34,25.27 13.08,25.02 | 13.34,25.27 13.59,25.02
A3  (via drill 0.3 pad 0.64)
  Top 0.203: U2.26 33.81,25.94 v32.51,24.64 | A2.2 11.25,12.9 v12.06,13.72 12.45,13.72 C53.1
  Bottom 0.203: v12.06,13.72 12.06,23.24 13.46,24.64 v32.51,24.64
D0  (via drill 0.3 pad 0.64)
  Top 0.203: U2.30 37.01,26.23 38.23,25.02 v38.23,23.88 | SERIAL.1 34.79,12.82 C33.1 34.92,13.72 v34.8,13.84
  Bottom 0.203: v34.8,13.84 34.8,20.45 v38.23,23.88
D1  (via drill 0.3 pad 0.64)
  Top 0.203: U2.31 37.81,26.19 39.12,24.89 v39.12,24.13 | 32.77,9.78 32.89,9.91 | 32.89,9.91 SERIAL.2 | 32.77,9.91 SERIAL.2 | SERIAL.2 | 32.89,9.91 32.89,12.45 C34.1 v33.4,13.84
  Bottom 0.203: v39.12,24.13 39.12,23.62 35.56,20.07 35.56,13.72 35.05,13.21 34.04,13.21 v33.4,13.84
D2  (via drill 0.3 pad 0.64)
  Top 0.203: D2.1 49.09,12.64 C35.1 v49.4,13.84 | U2.32 38.61,26.16 40.51,24.26 v40.51,24.13
  Bottom 0.203: v40.51,24.13 40.51,18.67 45.97,13.21 48.77,13.21 v49.4,13.84
D3  (via drill 0.3 pad 0.64)
  Top 0.203: U2.1 40.9,28.57 41.27,28.19 v41.27,23.62 | D2.2 47.09,12.22 C36.1 v46.35,13.84 | D3.1 68.23,12.42 C37.1 v67.69,13.78
  Bottom 0.203: v41.27,23.62 41.27,19.07 45.74,14.61 46.1,14.61 | 46.1,14.61 46.35,14.61 | 46.35,14.61 46.61,14.61 | 46.61,14.61 64.01,14.61 65.66,12.95 66.86,12.95 v67.69,13.78 | v46.35,13.84 46.35,14.35 | 46.35,14.35 46.35,14.61 | 46.35,14.35 46.1,14.61 | 46.35,14.35 46.61,14.61
D4  (via drill 0.3 pad 0.64)
  Top 0.203: U2.2 41.12,29.37 41.91,28.57 v41.91,24.13 | D3.2 66.23,12.89 C38.1 66.17,13.72 v66.1,13.78 | v83.44,13.84 C39.1 83.05,12.57 D4.1
  Bottom 0.203: v41.91,24.13 41.91,19.18 45.85,15.24 65.91,15.24 | 65.91,15.24 66.04,15.24 | 66.04,15.24 66.29,15.24 | v66.1,13.78 66.1,15.05 | 66.1,15.05 66.1,15.18 66.04,15.24 | 66.1,15.05 65.91,15.24 | 66.1,15.05 66.29,15.24 | 66.29,15.24 75.06,15.24 77.22,13.08 82.68,13.08 v83.44,13.84
D5  (via drill 0.3 pad 0.64)
  Top 0.203: U2.9 38.61,36.47 40.5,38.35 v42.04,38.35 | v58.8,40.26 C41.1 60.02,40.72 D5.1 67.23,40.72 69.85,38.1 v69.85,23.11 | D4.2 81.05,12.29 C40.1 v80.39,13.84
  Bottom 0.203: v42.04,38.35 42.04,40.18 42.76,40.89 58.17,40.89 v58.8,40.26 | v69.85,23.11 69.85,21.12 77.13,13.84 v80.39,13.84
D6  (via drill 0.3 pad 0.64)
  Top 0.203: U2.10 37.81,36.52 40.22,38.92 v43.05,38.92 | D6.1 59.99,24.84 C43.1 v58.8,25.27 | v58.8,38.73 C42.1 59.58,38.72 D5.2
  Bottom 0.203: v58.8,25.27 v58.8,38.73 58.17,39.37 43.43,39.37 43.05,38.99 v43.05,38.92
D7  (via drill 0.3 pad 0.64)
  Top 0.203: U2.11 37.01,36.62 39.76,39.37 42.55,39.37 43.09,39.91 v43.09,40.26 41.91,41.44 41.91,44.32 42.42,44.83 C45.1 43.09,44.87 D7.1 | D6.2 60.18,22.84 C44.1 58.77,22.23 58.32,22.67 v58.32,24.41
  Bottom 0.203: v43.09,40.26 57.91,40.26 58.67,39.5 59.05,39.5 59.56,38.99 59.56,25.02 58.95,24.41 v58.32,24.41
D8  (via drill 0.3 pad 0.64)
  Top 0.203: U2.12 36.21,38.12 38.23,40.13 v38.23,44.45 | v57.91,44.83 C47.1 59.56,45.85 60.07,46.35 61.98,46.35 62.23,46.61 D8.1 | v44.32,45.09 44.58,44.83 C46.1 D7.2
  Bottom 0.203: v57.91,44.83 44.58,44.83 v44.32,45.09 38.86,45.09 v38.23,44.45
D9  (via drill 0.3 pad 0.64)
  Top 0.203: U2.13 35.41,33.89 v35.31,33.78 | D8.2 64.23,46.45 62.61,44.83 C48.1 v61.09,45.72
  Bottom 0.203: v35.31,33.78 38.23,36.7 38.23,37.59 44.7,44.07 59.44,44.07 v61.09,45.72
GND  (via drill 0.3 pad 0.64)
  Top 0.203: v38.23,38.73 39.24,39.75 40.13,39.75 41.27,40.89 41.27,43.12 v41.21,43.18
  Top 0.305: U6.18 23.77,33 23.5,33.27 23.5,34.16 23.62,34.29 v23.69,34.29 | C12.2 29.71,33.52 29.97,33.78 29.97,34.16 30.1,34.16
  Top 0.356: C5.2 16.76,32.13 17.63,33 U6.3 19.6,33 v19.75,33.15 v19.75,34.42 19.63,34.3 U6.1 | U6.20 v23.69,34.3 v23.69,34.29 | U6.18 26.12,33 v26.61,32.51 26.67,32.45 26.67,32.26 26.9,32.03 C1.1
  other vias: 7.87,30.73 7.87,17.02 15.24,7.87 78.23,17.4 78.23,32.13 62.36,33.53 62.36,17.78 69.34,47.88 78.23,46.35 50.16,47.88 30.23,36.83 30.23,35.05 11.56,30.73 36.58,16.64 44.58,31.37 46.23,31.37 42.86,36.2 43.88,37.21 44.96,38.48 43.81,32.38 42.29,32.38 40.7,36.2 40.7,35.05 48.77,31.37 51.31,31.37 47.5,31.37 50.04,31.37 51.31,32.64 51.31,33.91 50.04,33.91 48.77,33.91 48.77,35.18 50.04,35.18 51.31,35.18 51.31,36.45 46.23,38.48 47.5,38.48 48.77,38.48 50.04,38.48 51.31,38.48 38.93,31.75 38.93,30.61 30.04,34.16 27.62,27.94 25.34,27.94 16.07,31.24 2.54,31.75 12.95,18.16 27.81,12.95 43.31,11.94 76.33,12.95 74.93,17.91 75.69,32.64 75.95,47.5 49.72,45.53 33.08,51.05 2.54,45.09 2.54,34.42 2.54,23.11 2.54,18.16 2.54,9.65 13.97,2.54 22.61,2.54 28.57,7.87 27.43,2.54 36.07,2.54 41.78,2.54 43.05,7.87 62.23,7.87 60.96,2.54 50.42,2.54 76.83,7.87 75.69,2.54 84.33,2.54 85.72,15.11 85.72,25.91 85.72,31.88 85.72,40.51 85.72,46.1 85.72,54.74 69.47,55.24 50.29,55.24 39.5,55.24 65.41,42.16 66.17,30.1 67.31,27.56 67.31,16 69.47,2.54 60.45,33.91 59.44,17.91 43.69,27.56 42.55,28.07 67.44,21.97 64.64,19.56 56.52,18.03 48.26,21.97 33.66,21.59 30.99,21.59 31.5,15.37 63.88,16 56.52,16 64.64,22.1 75.95,41.4 72.9,50.29 72.14,48.9 65.41,45.09 69.85,46.35 68.07,44.32 69.22,42.16 76.07,15.88 81.92,13.84 56.39,38.73 52.45,42.55 53.59,45.47 45.72,45.72 45.72,43.18 29.84,16.51 16.45,34.8 16.13,47.12 16.13,48.9 8.89,46.35 4.45,46.35 0.76,47.62 29.21,38.35 19.3,38.23 22.48,21.46 67.44,17.78 14.48,38.67 17.4,46.1 8.89,50.67 4.45,50.67 51.44,27.3 60.33,27.56 56.77,27.3 51.44,24.26 57.23,25.97 63.88,27.43 70.87,25.53 71.12,32.38 71.12,36.32 66.42,39.62 56.13,41.78 31.43,27.43 25.46,24 22.48,24 32.7,30.86 35.75,30.86 38.73,34.29 38.8,28.57 23.5,38.35 25.4,38.35 23.5,40.89 24.77,50.16 21.59,50.16 21.59,45.21 24.77,48.26 36.2,50.16 36.2,46.35 46.35,55.24 65.41,55.24 82.55,48.26 82.55,34.29 83.19,22.86 80.64,4.45 78.11,4.45 67.31,4.45 64.01,4.45 48.26,4.45 44.45,4.45 33.66,4.45 29.84,4.45 20.32,4.45 15.88,4.45 4.45,12.7 4.45,16.51 4.45,24.77 4.45,29.84 4.45,37.47 4.45,42.55 83.19,19.68 82.55,39.37 82.55,53.34 42.55,52.7 48.26,52.7 61.59,52.7 67.31,52.7 51.31,37.47 15.37,14.22 15.75,12.06 14.35,11.81 20.45,13.84 23.5,13.84 31.88,12.06 62.1,43.31 58.67,43.31 58.67,41.91 60.45,37.72 75.95,23.75 76.07,26.8 84.96,13.84 70.42,12.95 65.21,12.06 61.72,12.06 50.93,13.78 47.94,12.06 36.45,13.84 12.95,21.34 11.94,25.4 11.94,35.69 11.94,38.73 11.94,43.43 75.95,52.2 75.95,55.24 60.58,23.75 14.73,36.83 46.35,19.05 57.78,33.02 70.48,19.05 70.48,22.23 43.18,24.13 29.84,25.91 18.67,16.89 16.26,17.02 31.11,45.09 29.21,42.55 32.38,38.35 23.69,27.94 32,35.05 55.5,37.34 55.5,34.04
  pour Top (isolate 0.254): -0.64,58.42 88.27,58.42 88.27,-0.64 -0.64,-0.64
  pour Bottom (isolate 0.254): -0.64,58.42 88.27,58.42 88.27,-0.64 -0.64,-0.64
MCUVIN  (via drill 0.3 pad 0.64)
  Top 0.508: U2.4 41.42,30.97 41.47,30.92 | U2.6 40.96,32.57 41.4,32.13 41.4,31.24 | 41.4,30.99 41.4,31.24 | 41.4,31.24 41.15,30.99
  Top 0.61: L1.2 C8.1 42.8,30.35 C2.1 v41.91,30.48 41.47,30.92 41.4,30.99 | L19.1 27.3,30.48 v26.67,29.84
  Bottom 0.508: v26.67,29.84 41.27,29.84 v41.91,30.48
MISO  (via drill 0.3 pad 0.64)
  Top 0.203: U6.16 23.17,31.7 v22.99,31.88 | U2.16 v33.02,34.67
  Bottom 0.203: v22.99,31.88 30.23,31.88 v33.02,34.67 34.42,36.07 ISP.1
MOSI  (via drill 0.3 pad 0.64)
  Top 0.203: U2.15 33.81,37.05 v33.78,37.08 35.81,39.12 35.81,42.29 ISP.5 | U6.17 23.41,32.35 v22.99,32.77
  Bottom 0.203: v22.99,32.77 23.37,33.15 29.84,33.15 31.24,34.54 31.24,35.18 33.15,37.08 v33.78,37.08
N$1
  Top 0.305: R5.1 43.88,34.29 R1.1 43.94,36.07 44.95,37.07 X1.1 48.15,37.07 C3.1
N$2
  Top 0.203: R3.2 PWR.+
N$3
  Top 0.305: R4.1 43.88,33.27 R1.2 45.64,33.34 X1.2 48.88,32.75 48.9,32.77 C4.1
N$4
  Top 0.508: U2.18 30.57,33.37 29.23,32.03 C1.2 29.11,30.5 L19.2
N$17
  Top 0.203: RST.+ 30.97,20.25 R2.2
N$19  (via drill 0.3 pad 0.64)
  Top 0.61: v15.88,50.55 12.06,50.55 L3.1 4.57,49.15 2.62,51.1 RPI_COON.1
  Bottom 0.61: v15.88,50.55 20.7,50.55 RPI_COON.17
N$20
  Top 0.203: U2.20 30.73,31.77 30.23,31.26 30.23,29.46 29.69,28.93 C6.2
N$21  (via drill 0.3 pad 0.64)
  Top 0.61: v12.19,48.9 v12.19,48.26
  Top 1.27: L2.1 C14.1 13.21,47.24 C13.1 v12.19,48.9
  Bottom 1.27: RPI_COON.4 RPI_COON.2 1.98,55.32 0.95,54.29 0.95,50.42 1.02,50.42 2.92,48.51 11.81,48.51 v12.19,48.9
N$22
  Top 0.305: U2.8 41.85,34.17 R5.2 C30.2
N$23
  Top 0.305: U2.7 41.88,33.37 R4.2
RESET  (via drill 0.3 pad 0.64)
  Top 0.203: U2.29 36.21,25.55 R6.1 34.93,24.39 34.93,24.26 34.54,23.88 v31.75,23.88 27.05,23.88 26.04,24.89 26.04,30.1 25.72,30.41 U6.14 23.3,30.41 v22.99,30.1 | RST.- v31.74,16.64 v31.75,16.64
  Bottom 0.203: ISP.3 37.59,38.99 37.59,37.08 v34.16,33.66 30.99,30.48 23.37,30.48 v22.99,30.1 | v31.75,16.64 v31.75,23.88
RPI-RX  (via drill 0.3 pad 0.64)
  Top 0.203: U6.9 17.67,29.1 17.27,28.7 v17.27,27.94
  Bottom 0.203: RPI_COON.10 12.78,55.3 14.1,53.98 14.1,50.16 13.72,49.78 13.72,44.07 14.99,42.8 14.99,40.01 13.72,38.73 13.72,31.88 17.27,28.32 v17.27,27.94
RPI-SCL
  Top 0.203: R7.1 28.54,47.98 Q4.2 28.37,48.08 27.43,49.02 19.94,49.02 17.27,51.69 8.76,51.69 7.7,52.76 RPI_COON.5
RPI-SDA
  Top 0.203: R9.1 20.33,48 Q5.2 19.81,48.51 19.68,48.51 16.89,51.31 6.6,51.31 5.16,52.76 RPI_COON.3
RPI-TX  (via drill 0.3 pad 0.64)
  Top 0.203: U6.8 16.92,29.75 16.38,29.21 v16.38,27.94
  Bottom 0.203: RPI_COON.8 10.24,55.3 11.56,53.98 11.56,51.31 13.21,49.66 13.21,43.94 14.48,42.67 14.48,40.13 13.21,38.86 13.21,31.62 16.38,28.45 v16.38,27.94
RPI_MISO  (via drill 0.3 pad 0.64)
  Top 0.203: U6.5 20.27,31.7 v20.45,31.88
  Bottom 0.203: v20.45,31.88 21.08,32.51 21.08,42.16 23.62,44.7 28.07,44.7 28.83,45.47 28.83,51.97 RPI_COON.21
RPI_MOSI  (via drill 0.3 pad 0.64)
  Top 0.203: U6.4 20.03,32.35 v20.45,32.77
  Bottom 0.203: v20.45,32.77 20.45,42.29 23.5,45.34 27.94,45.34 28.32,45.72 28.32,49.94 RPI_COON.19
RPI_RESET  (via drill 0.3 pad 0.64)
  Top 0.203: U6.7 20.15,30.4 v20.45,30.1
  Bottom 0.203: v20.45,30.1 21.97,31.62 21.97,41.66 24,43.69 28.45,43.69 29.97,45.21 29.97,49.78 31.88,51.69 31.88,54 RPI_COON.24
RPI_SCK  (via drill 0.3 pad 0.64)
  Top 0.203: U6.6 20.39,31.05 v20.45,30.99
  Bottom 0.203: v20.45,30.99 21.59,32.13 21.59,41.91 23.88,44.2 28.19,44.2 29.34,45.34 29.34,51.56 RPI_COON.23
RX  (via drill 0.3 pad 0.64)
  Top 0.203: U6.12 23.78,29.11 21.34,26.67 v21.34,23.88 | RPISER.1 21.27,12.26 C31.1 v21.97,13.84
  Bottom 0.203: v21.34,23.88 21.34,14.48 v21.97,13.84
SCK  (via drill 0.3 pad 0.64)
  Top 0.203: U6.15 23.05,31.05 v22.99,30.99 | U2.17 32.51,34.17 v33.02,33.66
  Bottom 0.203: v22.99,30.99 30.1,30.99 32.77,33.66 v33.02,33.66 36.96,37.59 ISP.2
SCL-BOARD  (via drill 0.3 pad 0.64)
  Top 0.203: Q4.3 26.4,44.45 R8.1 26.66,43.07 v26.67,43.05 | U2.28 35.41,28.18 v35.43,28.19 | v74.17,25.27 C60.1 75.56,24.64 I2C-3.1 | I2C-1.1 75.42,39.26 C56.1 v74.17,39.75 | I2C-2.1 75.23,53.42 C58.1 v74.17,53.72
  Bottom 0.203: v26.67,43.05 24,43.05 22.35,41.4 22.35,29.59 22.99,28.96 34.67,28.96 v35.43,28.19 34.42,27.18 34.42,26.16 34.67,25.91 54.86,25.91 57.66,23.11 61.47,23.11 62.48,24.13 73.03,24.13 v74.17,25.27 74.17,35.69 73.53,36.32 73.53,39.5 | 73.53,39.5 73.53,39.75 | 73.53,39.75 73.53,40.01 | 73.53,40.01 73.53,53.09 v74.17,53.72 | v74.17,39.75 73.79,39.75 | 73.79,39.75 73.53,39.75 | 73.79,39.75 73.53,40.01 | 73.79,39.75 73.53,39.5
SDA-BOARD  (via drill 0.3 pad 0.64)
  Top 0.203: Q5.3 18.16,44.55 R10.1 v18.41,43.44 v18.41,43.43 | U2.27 34.61,28 v34.42,28.19 | I2C-3.2 75.35,22.64 C59.1 v74.17,22.23 | v74.17,36.7 C55.1 75.49,37.26 I2C-1.2 | I2C-2.2 75.68,51.42 C57.1 v74.17,50.67
  Bottom 0.203: v18.41,43.43 18.41,31.24 21.08,28.57 34.04,28.57 v34.42,28.19 33.91,27.69 33.91,26.04 34.54,25.4 54.74,25.4 57.4,22.73 61.72,22.73 62.74,23.75 73.91,23.75 | v74.17,50.67 75.06,49.78 75.06,36.96 | 75.06,36.45 75.06,24.89 74.17,24 | 75.06,36.45 75.06,36.7 | 75.06,36.7 75.06,36.96 | v74.17,36.7 74.8,36.7 | 74.8,36.7 75.06,36.7 | 74.8,36.7 75.06,36.96 | 74.8,36.7 75.06,36.45 | 74.17,23.75 73.91,23.75 | v74.17,22.23 74.17,23.5 | 74.17,23.5 74.17,23.75 | 74.17,23.75 74.17,24 | 73.91,23.75 74.17,24 | 73.91,23.75 74.17,23.5
TX  (via drill 0.3 pad 0.64)
  Top 0.203: U6.13 23.67,29.76 20.45,26.54 v20.45,23.88 | RPISER.2 19.3,9.93 19.3,12.57 C32.1 v18.92,13.84
  Bottom 0.203: v20.45,23.88 20.45,15.37 v18.92,13.84
(copper drawn outside any net)
  shapes: Bottom circle x1

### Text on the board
Bottom: B
bPlace: GrovePi+ | by Dexter Industries / and Seeed Studio | v3.0 01/11/2016
_tsilk: U$15 | I2C-1 | Q4 | Q5 | R7 | R9 | D7 | D8 | R10 | A0 | R8 | J12 | C11 | I2C-2 | C5 | D6 | Y1 | C10 | A1 | U1 | C12 | U6 | I2C-3 | R6 | GrovePi V2 | R2 | R3 | D5 | GrovePi V2 | RST | PWR | A2 | PI-SER | SERIAL | D2 | D3 | D4

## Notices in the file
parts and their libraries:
moudle-new: This work is licensed under the Creative Commons Attribution 4.0 International License.
To view a copy of this license,visit:
http://creativecommons.org/licenses/by-sa/4.0
moudle-new: CC-BY-SA
